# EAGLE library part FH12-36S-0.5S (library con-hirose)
0.5mm Pitch Connectors For FPC/FFC Source: Data sheet
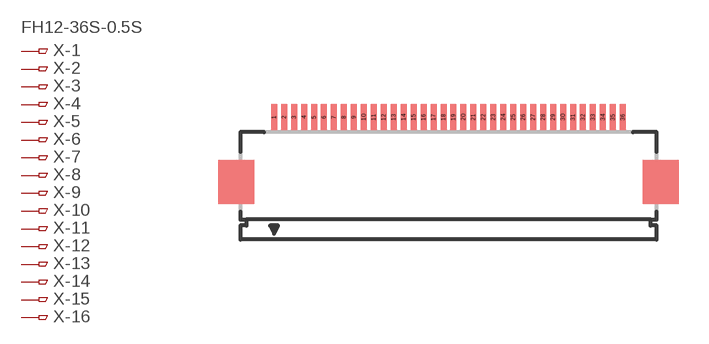
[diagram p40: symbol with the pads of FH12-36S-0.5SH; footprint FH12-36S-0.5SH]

Designator prefix X; gates -1=PINV -2=PIN -3=PIN -4=PIN -5=PIN -6=PIN -7=PIN -8=PIN -9=PIN -10=PIN -11=PIN -12=PIN -13=PIN -14=PIN -15=PIN -16=PIN -17=PIN -18=PIN -19=PIN -20=PIN -21=PIN -22=PIN -23=PIN -24=PIN -25=PIN -26=PIN -27=PIN -28=PIN -29=PIN -30=PIN -31=PIN -32=PIN -33=PIN -34=PIN -35=PIN -36=PIN

## FH12-36S-0.5SH (OC_FARNELL: unknown; OC_NEWARK: unknown)  [FH12-36S-0.5SH]
1  -1:1  pas
2  -2:1  pas
3  -3:1  pas
4  -4:1  pas
5  -5:1  pas
6  -6:1  pas
7  -7:1  pas
8  -8:1  pas
9  -9:1  pas
10  -10:1  pas
11  -11:1  pas
12  -12:1  pas
13  -13:1  pas
14  -14:1  pas
15  -15:1  pas
16  -16:1  pas
17  -17:1  pas
18  -18:1  pas
19  -19:1  pas
20  -20:1  pas
21  -21:1  pas
22  -22:1  pas
23  -23:1  pas
24  -24:1  pas
25  -25:1  pas
26  -26:1  pas
27  -27:1  pas
28  -28:1  pas
29  -29:1  pas
30  -30:1  pas
31  -31:1  pas
32  -32:1  pas
33  -33:1  pas
34  -34:1  pas
35  -35:1  pas
36  -36:1  pas

## Footprint FH12-36S-0.5SH (pad centres in mm)
0.5mm Pitch Connectors For FPC/FFC Source: Data sheet
smd 0.3 x 1.3: 1 -8.75,3.25; 2 -8.25,3.25; 3 -7.75,3.25; 4 -7.25,3.25; 5 -6.75,3.25; 6 -6.25,3.25; 7 -5.75,3.25; 8 -5.25,3.25; 9 -4.75,3.25; 10 -4.25,3.25; 11 -3.75,3.25; 12 -3.25,3.25; 13 -2.75,3.25; 14 -2.25,3.25; 15 -1.75,3.25; 16 -1.25,3.25; 17 -0.75,3.25; 18 -0.25,3.25; 19 0.25,3.25; 20 0.75,3.25; 21 1.25,3.25; 22 1.75,3.25; 23 2.25,3.25; 24 2.75,3.25; 25 3.25,3.25; 26 3.75,3.25; 27 4.25,3.25; 28 4.75,3.25; 29 5.25,3.25; 30 5.75,3.25; 31 6.25,3.25; 32 6.75,3.25; 33 7.25,3.25; 34 7.75,3.25; 35 8.25,3.25; 36 8.75,3.25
